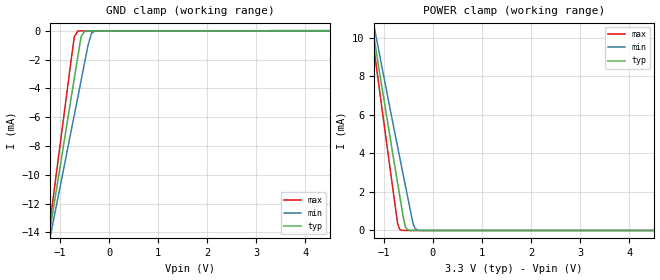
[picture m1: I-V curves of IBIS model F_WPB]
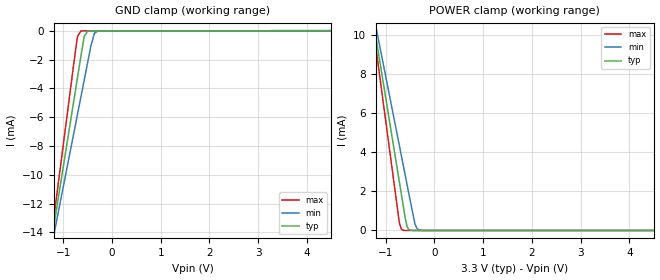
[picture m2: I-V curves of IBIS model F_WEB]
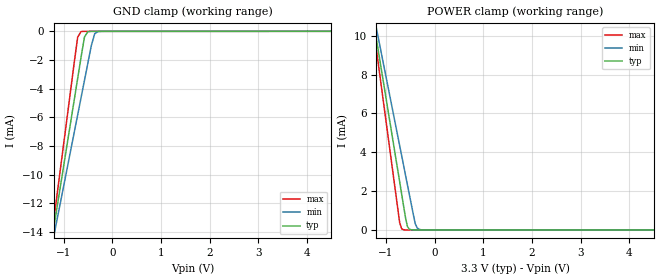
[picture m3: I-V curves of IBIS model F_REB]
| This IBIS file was created by s2ibis3 version 1.1
| North Carolina State University, ERL, 2006
[IBIS ver] 3.2
[File name] s34sl01g2_a_i_33_r1.ibs
[File Rev] 1.0
| Rev 1.0 - 07/08/2015 - Initial IBIS model created (x8 ONFI)
[Date]  08/14/2015
[Source] File generated by Cypress IBIS Team
[Notes]  Generated IBIS models from SPICE simulations.
|   This model containts package model and model selector statements
|   It is require to select appropriate package model and driver for each
|   paths such as NAND and SNAND. Please select NAND package model for
|   NAND path simulations and SNAND package model for SNAND simulations.
|   - Voltage condition is [3.3V  2.7V  3.6V]
|   - Temperature condition is [25C  85C  -40C]
[Disclaimer] THE MODEL LIBRARIES ARE PROVIDED AS IS.
[Copyright] (C) COPYRIGHT 2015
| CYPRESS
| ALL RIGHTS RESERVED.
|   Component u796 (SNAND + 1G NAND in 63 BALL package)
[Component] U796_MCP
[Manufacturer] CYPRESS
[Package]
| Package V2B063
| variable   typ   min   max
R_pkg   0.0   0.0   0.0
L_pkg   0.0H   0.0H   0.0H
C_pkg   0.0F   0.0F   0.0F
|Note: Since [Define package model] statement is present,
|   default package RLC values will not be used by IBIS simulation
|   and hence these values are set to zero (simply for model completion).
[Pin]   signal_name  model_name   R_pin   L_pin   C_pin
A1   NC   NC
A2   NC   NC
A9   NC   NC
A10   NC   NC
B1   NC   NC
B9   NC   NC
B10   NC   NC
C3   WP#   F_WPB
C4   ALE   ALE
C5   VSS   GND
C6   CE#   CEB
C7   WE#   WEB
C8   RB#   RBb_BUF
D3   VCC   POWER
D4   RE#   REB
D5   CLE   CLE
D6   NC   NC
D7   NC   NC
D8   NC   NC
E3   NC   NC
E4   NC   NC
E5   NC   NC
E6   NC   NC
E7   NC   NC
E8   NC   NC
F3   NC   NC
F4   NC   NC
F5   NC   NC
F6   NC   NC
F7   VSS   GND
F8   NC   NC
G3   NC   NC
G4   VCC   POWER
G5   VPE   F_VPE
G6   NC   NC
G7   NC   NC
G8   NC   NC
H3   NC   NC
H4   I/O0   DQ
H5   NC   NC
H6   NC   NC
H7   NC   NC
H8   VCC   POWER
J3   NC   NC
J4   I/O1   DQ
J5   NC   NC
J6   VCC   POWER
J7   I/O5   DQ
J8   I/O7   DQ
K3   VSS   GND
K4   I/O2   DQ
K5   I/O3   DQ
K6   I/O4   DQ
K7   I/O6   DQ
K8   VSS   GND
L1   NC   NC
L2   NC   NC
L9   NC   NC
L10   NC   NC
M1   NC   NC
M2   NC   NC
M9   NC   NC
M10   NC   NC
|[Package Model] U796_SNAND
|If user simulation tool cannot handle [Alternate package models] keyword,
|please comment out that keyword and substatements.
[Alternate Package Models]
U796_snand |choose this package model to evaluate SNAND signal paths
U796_nand  |choose this package model to evaluate NAND signal paths
[End Alternate Package Models]
|SNAND package paths modelled
[Define Package Model]  U796_snand
[Manufacturer]   CYPRESS
[OEM]   n/a
[Description]   11033A_SNAND_33V
[Number Of Pins]   16
[Pin Numbers]
|[Pin Name]  Net Number   Net Name   Net's All Pins
D3   | 1   VCC   D3
   |G4
   |H8
   |J6
C4   | 2   ALE   C4
C6   | 3   CE#   C6
D5   | 4   CLE   D5
H4   | 5   IO0   H4
J4   | 6   IO1   J4
K4   | 7   IO2   K4
K5   | 8   IO3   K5
K6   | 9   IO4   K6
J7   | 10   IO5   J7
K7   | 11   IO6   K7
J8   | 12   IO7   J8
D4   | 13   RE#   D4
G5   | 14   VPE   G5
C7   | 15   WE#   C7
C3   | 16   WP#   C3
[Model Data]
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[End Model Data]
[End Package Model]
|NAND package paths modelled
[Define Package Model]   U796_1g_nand
[Manufacturer]   CYPRESS
[OEM]   n/a
[Description]   98663A1_1G_NAND
[Number of Pins]   15
[Pin Numbers]
|[Pin Name]  Net Number   Net Name   Net's All Pins
D3   | 1   VCC   D3
   |G4
   |H8
   |J6
C4   | 2   ALE   C4
C6   | 3   CE#   C6
D5   | 4   CLE   D5
H4   | 5   IO0   H4
J4   | 6   IO1   J4
K4   | 7   IO2   K4
K5   | 8   IO3   K5
K6   | 9   IO4   K6
J7   | 10   IO5   J7
K7   | 11   IO6   K7
J8   | 12   IO7   J8
C8   | 13   RB#   C8
D4   | 14   RE#   D4
C7   | 15   WE#   C7
[Model Data]
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[End Model Data]
[End Package Model]
| Model Selector
[Model Selector] WEB
F_WEB   SNAND IO Driver
IN_CTL   NAND input buffer
[Model Selector] REB
F_REB   SNAND IO Driver
IN_CTL   NAND input buffer
[Model Selector] ALE
F_ALE   SNAND IO Driver
IN_CTL   NAND input buffer
[Model Selector] CLE
F_CLE   SNAND IO Driver
IN_CTL   NAND input buffer
[Model Selector] CEB
F_CEB   SNAND IO Driver
IN_CTL   NAND input buffer
[Model Selector] DQ
F_DQ   SNAND IO Driver
DQ_BUF   NAND IO Driver
| Models and submodels in the file (11): F_WPB (Input), F_WEB (Input), F_REB (Input), F_ALE (Input), F_CLE (Input), F_VPE (Input), F_CEB (Input), F_DQ (I/O), IN_CTL (Input), DQ_BUF (I/O), RBb_BUF (Open_drain)
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|Driver/receiver models for SNAND component of MCP
|   Model   F_WPB
[Model]   F_WPB
Model_type Input
Vinl =   0.6600V
Vinh =   2.6400V
   C_comp   1.3833pF   1.3743pF   1.3881pF
[Temperature Range]   25.0000   0.1050k   -40.0000
[Pullup Reference]   3.3000V   3.0000V   3.6000V
[Pulldown Reference]   0.0V   0.0V   0.0V
[POWER Clamp Reference]   3.3000V   3.0000V   3.6000V
[GND Clamp Reference]   0.0V   0.0V   0.0V
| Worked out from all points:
|   GND clamp passes 1 mA (typ) near -0.60 V on its own axis
|   POWER clamp passes 1 mA (typ) near -0.62 V on its own axis
[GND_clamp]
|Voltage   I(typ)   I(min)   I(max)
-3.3V     -58.25mA   -50.51mA   -68.01mA
-1.27V    -15.17mA   -15.49mA   -14.97mA
-1.2V     -13.69mA   -14.29mA   -13.14mA
-1.13V    -12.2mA    -13.08mA   -11.31mA
-710mV    -3.287mA   -5.833mA   -407.1uA
-640mV    -1.802mA   -4.625mA   -14.79uA
-570mV    -392.7uA   -3.418mA   -1.334uA
-500mV    -28.41uA   -2.21mA    -916.6nA
-430mV    -2.329uA   -1.003mA   -902.8nA
-360mV    -604.8nA   -162.9uA   -902.3nA
-290mV    -490.1nA   -19.76uA   -902.2nA
6.6V      39.72pA    16.99uA    -233.3nA
[POWER_clamp]
|Voltage   I(typ)   I(min)   I(max)
-3.28V    42.98mA    38.08mA    49.06mA
-1.28V    11.24mA    11.65mA    10.92mA
-1.24V    10.61mA    11.12mA    10.16mA
-1.2V     9.976mA    10.6mA     9.399mA
-1.16V    9.344mA    10.07mA    8.639mA
-720mV    2.468mA    4.337mA    379.5uA
-680mV    1.854mA    3.828mA    64.23uA
-640mV    1.24mA     3.32mA     9.947uA
-560mV    171.1uA    2.309mA    809.7nA
-400mV    603.9nA    322.6uA    371.8nA
-280mV    161.8nA    9.267uA    251.9nA
6.6V      39.72pA    2.996nA    43.19pA
|   Model   F_WEB
[Model]   F_WEB
Model_type Input
Vinl =   0.6600V
Vinh =   2.6400V
   C_comp   1.3359pF   1.3158pF   1.3470pF
[Temperature Range]   25.0000   0.1050k   -40.0000
[Pullup Reference]   3.3000V   3.0000V   3.6000V
[Pulldown Reference]   0.0V   0.0V   0.0V
[POWER Clamp Reference]   3.3000V   3.0000V   3.6000V
[GND Clamp Reference]   0.0V   0.0V   0.0V
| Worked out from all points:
|   GND clamp passes 1 mA (typ) near -0.60 V on its own axis
|   POWER clamp passes 1 mA (typ) near -0.62 V on its own axis
[GND_clamp]
|Voltage   I(typ)   I(min)   I(max)
-3.3V     -58.25mA   -50.51mA   -68.01mA
-1.27V    -15.17mA   -15.49mA   -14.97mA
-1.2V     -13.69mA   -14.29mA   -13.14mA
-1.13V    -12.2mA    -13.08mA   -11.31mA
-710mV    -3.287mA   -5.833mA   -406.4uA
-640mV    -1.801mA   -4.625mA   -13.92uA
-570mV    -392.3uA   -3.417mA   -432.3nA
-500mV    -27.95uA   -2.21mA    -14.31nA
-430mV    -1.849uA   -1.002mA   -500.6pA
-360mV    -123.6nA   -162.7uA   -58.79pA
-290mV    -8.752nA   -19.51uA   -43.43pA
6.6V      39.73pA    16.96uA    36.6pA
[POWER_clamp]
|Voltage   I(typ)   I(min)   I(max)
-3.28V    41.85mA    36.71mA    48.13mA
-1.28V    11.09mA    11.42mA    10.82mA
-1.24V    10.47mA    10.92mA    10.07mA
-1.2V     9.856mA    10.41mA    9.323mA
-1.16V    9.241mA    9.904mA    8.577mA
-720mV    2.474mA    4.34mA     378.9uA
-680mV    1.859mA    3.834mA    63.12uA
-640mV    1.244mA    3.328mA    8.921uA
-560mV    171.5uA    2.316mA    167.4nA
-400mV    368.6nA    323.9uA    110.7pA
-280mV    3.503nA    9.212uA    50.14pA
6.6V      39.73pA    2.996nA    43.2pA
|   Model   F_REB
[Model]   F_REB
Model_type Input
Vinl =   0.6600V
Vinh =   2.6400V
   C_comp   1.3400pF   1.3198pF   1.3510pF
[Temperature Range]   25.0000   0.1050k   -40.0000
[Pullup Reference]   3.3000V   3.0000V   3.6000V
[Pulldown Reference]   0.0V   0.0V   0.0V
[POWER Clamp Reference]   3.3000V   3.0000V   3.6000V
[GND Clamp Reference]   0.0V   0.0V   0.0V
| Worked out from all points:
|   GND clamp passes 1 mA (typ) near -0.60 V on its own axis
|   POWER clamp passes 1 mA (typ) near -0.62 V on its own axis
[GND_clamp]
|Voltage   I(typ)   I(min)   I(max)
-3.3V     -58.25mA   -50.51mA   -68.01mA
-1.27V    -15.17mA   -15.49mA   -14.97mA
-1.2V     -13.69mA   -14.29mA   -13.14mA
-1.13V    -12.2mA    -13.08mA   -11.31mA
-710mV    -3.287mA   -5.833mA   -406.4uA
-640mV    -1.801mA   -4.625mA   -13.92uA
-570mV    -392.3uA   -3.417mA   -432.3nA
-500mV    -27.95uA   -2.21mA    -14.31nA
-430mV    -1.849uA   -1.002mA   -500.6pA
-360mV    -123.6nA   -162.7uA   -58.79pA
-290mV    -8.752nA   -19.51uA   -43.43pA
6.6V      39.73pA    16.96uA    36.6pA
[POWER_clamp]
|Voltage   I(typ)   I(min)   I(max)
-3.28V    41.85mA    36.71mA    48.13mA
-1.28V    11.09mA    11.42mA    10.82mA
-1.24V    10.47mA    10.92mA    10.07mA
-1.2V     9.856mA    10.41mA    9.323mA
-1.16V    9.241mA    9.904mA    8.577mA
-720mV    2.474mA    4.34mA     378.9uA
-680mV    1.859mA    3.834mA    63.12uA
-640mV    1.244mA    3.328mA    8.921uA
-560mV    171.5uA    2.316mA    167.4nA
-400mV    368.6nA    323.9uA    110.7pA
-280mV    3.503nA    9.212uA    50.14pA
6.6V      39.73pA    2.996nA    43.2pA
